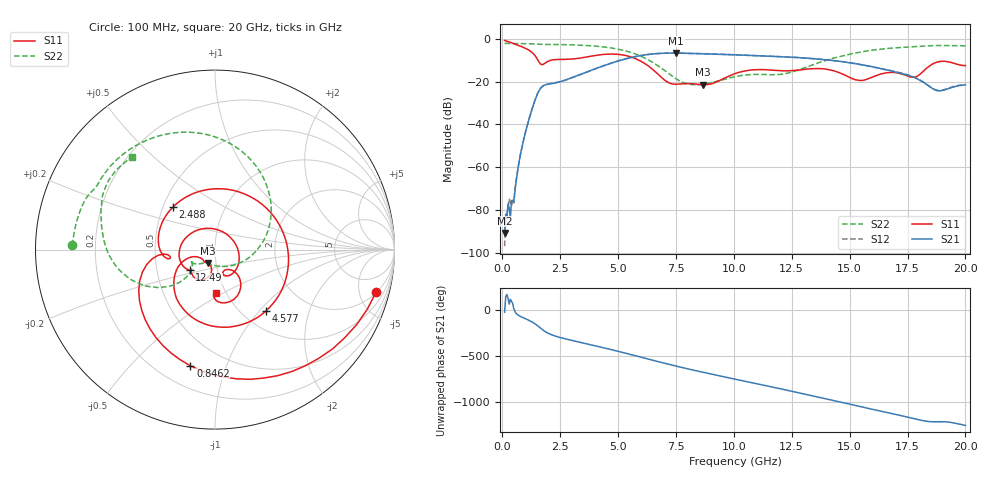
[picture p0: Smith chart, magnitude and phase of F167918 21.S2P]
!  2-Port S-parameters saved by WinCal
! VAR MeasName=S-Parameters (CALIBRATED_DATA) read from VNA (N5242A)
! VAR MeasDate=2016-11-22 10:25:46
! VAR NAME=F167918 21
! VAR FILENAME=F167918 21.S2P
! VAR DATE=2016-11-22 10:25:46
! VAR PHYS_PORTS=1,2
# Hz S DB R 50
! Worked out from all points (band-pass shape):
!   401 points, 100 MHz to 20 GHz, reference 50 ohm
!   highest |S21| = -6.56 dB at 7.513 GHz (marker M1); lowest = -90.9 dB at 100 MHz (marker M2)
!   |S21| within 3 dB of the highest: 5.238 GHz to 13.82 GHz (8.579 GHz wide, 90 % of centre)
!   lowest |S11| = -21.4 dB at 8.657 GHz (marker M3), VSWR 1.19, Z = 45.5 - j6.78 ohm
!   |S11| at or under -10 dB: 1.545 GHz to 2.074 GHz (529.2 MHz wide, 29.2 % of centre); 5.918 GHz to end of sweep
!   |S22| runs from -21.4 to -2.0 dB; largest |S21 - S12| = 0.005
!   S11 on the Smith chart (normalised r, x): 100 MHz: 2.08, -7.12; 846.2 MHz: 0.33, -0.76; 2.488 GHz: 0.56, +0.30; 4.577 GHz: 1.28, -1.09; 12.49 GHz: 0.74, -0.18; 20 GHz: 0.90, -0.46
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1e8  -0.65 -14.8  -90.85 -25.8  -97.00 71.5  -2.00 178.3
4.4825e8  -1.91 -57.8  -75.84 68.9  -74.69 12.1  -2.05 172.7
8.4625e8  -3.58 -102.0  -50.80 -79.9  -50.74 -78.2  -2.11 166.3
1.24425e9  -5.88 -145.9  -34.27 -125.8  -34.21 -125.6  -2.20 159.7
1.5925e9  -10.86 -175.0  -24.07 173.5  -24.01 173.4  -2.43 154.1
2.488e9  -9.55 134.5  -19.99 61.1  -19.95 60.8  -2.56 140.4
3.43325e9  -8.78 43.8  -16.35 4.5  -16.35 4.4  -2.89 121.5
4.03025e9  -7.67 -8.0  -13.84 -29.8  -13.83 -29.7  -3.31 107.1
4.5775e9  -7.05 -50.3  -11.73 -62.3  -11.70 -62.3  -3.96 91.6
5.72175e9  -8.99 -125.3  -8.27 -134.3  -8.23 -134.4  -6.88 49.9
6.7665e9  -16.88 -162.7  -6.74 157.6  -6.74 157.4  -12.84 -2.3
7.51275e9  -21.15 -138.4  -6.56 111.3  -6.57 111.2  -18.61 -52.5
8.657e9  -21.42 -119.4  -6.83 45.9  -6.83 45.8  -21.15 -120.7
1.005e10  -16.19 -103.3  -7.35 -29.5  -7.35 -29.4  -17.65 -142.4
1.1244e10  -14.29 -127.6  -7.90 -92.5  -7.88 -92.3  -16.54 -154.1
1.248775e10  -14.79 -140.6  -8.49 -158.8  -8.48 -158.9  -15.50 -140.4
1.338325e10  -13.91 -156.7  -9.13 151.9  -9.11 151.9  -12.13 -136.6
1.527375e10  -19.09 80.1  -11.55 45.6  -11.57 45.4  -6.46 -157.6
1.67165e10  -15.67 -51.0  -14.67 -35.1  -14.65 -34.4  -4.33 178.7
1.7811e10  -17.86 -60.2  -18.04 -97.7  -17.95 -97.2  -3.54 162.7
1.8806e10  -10.69 -67.1  -24.21 -129.0  -24.01 -128.0  -3.02 147.5
2e10  -12.38 -88.8  -21.43 -169.2  -21.25 -169.1  -3.16 131.9
